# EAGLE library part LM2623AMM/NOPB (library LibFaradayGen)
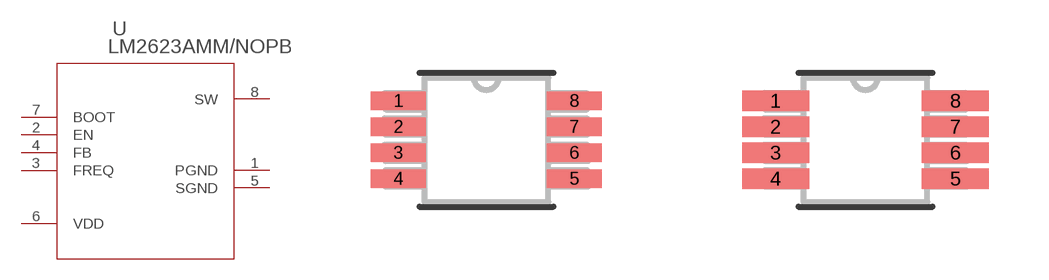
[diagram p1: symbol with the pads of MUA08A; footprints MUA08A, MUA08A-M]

Designator prefix U

## LM2623AMM/NOPB (MANUFACTURER_PART_NUMBER: LM2623AMMNOPB; VENDOR: Texas Instruments)  [MUA08A]
1  PGND  pas
2  EN  pas
3  FREQ  pas
4  FB  pas
5  SGND  pas
6  VDD  pas
7  BOOT  pas
8  SW  out

## LM2623AMM/NOPBMUA08A-M (MANUFACTURER_PART_NUMBER: LM2623AMMNOPB; VENDOR: Texas Instruments)  [MUA08A-M]
Pads as for MUA08A

## LM2623AMM/NOPBMUA08A-L (MANUFACTURER_PART_NUMBER: LM2623AMMNOPB; VENDOR: Texas Instruments)  [MUA08A-L]
Pads as for MUA08A

## Footprint MUA08A (pad centres in mm)
smd 1.372 x 0.457: 1 -2.197,0.975; 2 -2.197,0.325; 3 -2.197,-0.325; 4 -2.197,-0.975; 5 2.197,-0.975; 6 2.197,-0.325; 7 2.197,0.325; 8 2.197,0.975

## Footprint MUA08A-M (pad centres in mm)
smd 1.676 x 0.508: 1 -2.248,0.975; 2 -2.248,0.325; 3 -2.248,-0.325; 4 -2.248,-0.975; 5 2.248,-0.975; 6 2.248,-0.325; 7 2.248,0.325; 8 2.248,0.975

## Footprint MUA08A-L (pad centres in mm)
smd 1.067 x 0.406: 1 -2.146,0.975; 2 -2.146,0.325; 3 -2.146,-0.325; 4 -2.146,-0.975; 5 2.146,-0.975; 6 2.146,-0.325; 7 2.146,0.325; 8 2.146,0.975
